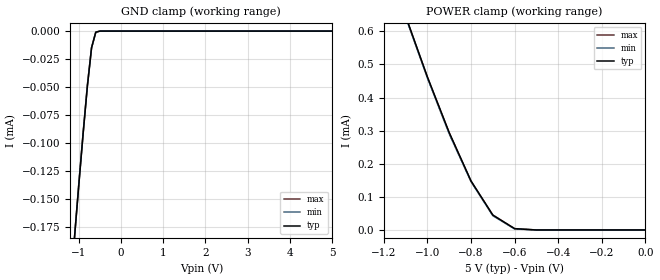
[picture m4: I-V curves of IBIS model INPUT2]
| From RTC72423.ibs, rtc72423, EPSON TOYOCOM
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[Model]   INPUT2
Model_type   Input
Polarity   Non-Inverting
Vinl =   1.0V
Vinh =   4.0V
C_comp   0.80pF   0.60pF   1.00pF
[Temperature Range]   25.00   85.00   -40.00
[Voltage Range]   5.0V   4.5V   5.50V
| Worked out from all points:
|   GND clamp passes 1 mA (typ) near -2.77 V on its own axis
|   POWER clamp passes 1 mA (typ) near -1.28 V on its own axis
[GND_clamp]
| voltage   I(typ)   I(min)   I(max)
-5V       -2.114mA   -2.114mA   -2.114mA
-1.1V     -183uA     -183uA     -183uA
-1V       -137uA     -136uA     -136uA
-900mV    -92uA      -91uA      -92uA
-800mV    -50uA      -49uA      -49uA
-700mV    -15uA      -15uA      -15uA
-600mV    -1uA       -1uA       -1uA
-500mV    0A         0A         0A
5V        0A         0A         0A
[POWER_clamp]
| voltage   I(typ)   I(min)   I(max)
-5V       8.995mA    8.999mA    9mA
-1.1V     646uA      643uA      645uA
-1V       462uA      459uA      461uA
-900mV    294uA      290uA      293uA
-800mV    148uA      146uA      147uA
-700mV    45uA       43uA       45uA
-600mV    4uA        3uA        4uA
-500mV    0A         0A         0A
0V        0A         0A         0A
